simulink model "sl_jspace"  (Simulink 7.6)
settings: Solver=ode45  StartTime=0.0  StopTime=10.0  RelTol=1e-3
libraries: roblocks x4, simulink x1

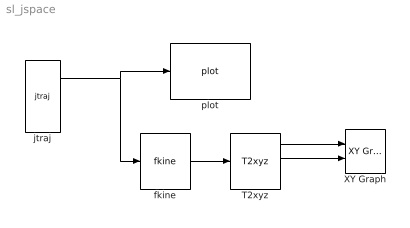
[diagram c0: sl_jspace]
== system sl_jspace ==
  T2xyz : roblocks/Transform Conversion/T2xyz  SystemSampleTime=-1
  XY Graph : simulink/Sinks/XY Graph  SystemSampleTime=-1  xmin=-1  xmax=1  ymin=-1  ymax=1  st=-1
  fkine : roblocks/Kinematics/fkine  SystemSampleTime=-1  robot=p560
  jtraj : roblocks/Trajectory/jtraj  SystemSampleTime=-1  q0=[0 0 0 0 0 0]  qf=[pi/4 pi/2 -pi/2 0 0 0]  tmax=10
  plot : roblocks/Robot Graphics/plot  SystemSampleTime=-1  robot=p560
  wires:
  jtraj/1 -> plot/1, fkine/1
  fkine/1 -> T2xyz/1
  T2xyz/1 -> XY Graph/1
  T2xyz/2 -> XY Graph/2
